| IBIS file stm32u3b5_3c5_wlcsp99_smps.ibs
[IBIS ver] 4.2
[File name] stm32u3b5_3c5_wlcsp99_smps.ibs
[File Rev] 0.1
[Date] 09-03-2026
[Source] Data Created at STMicroelectronics
[Notes]  File originated from ELDO simulations.
[Disclaimer]  This information is for modeling purpose only and is
   not guaranted. The information is subject to change without
   notice.
[Copyright] Copyright 2026 STMicroelectronics Inc.
|   Component stm32u3b5_3c5_wlcsp99_smps
[Component] stm32u3b5_3c5_wlcsp99_smps
[Manufacturer] STMicroelectronics
[Package]
| variable   typ   min   max
R_pkg  0  NA  NA
L_pkg  0  NA  NA
C_pkg  0  NA  NA
[Pin]   signal_name   model_name
A1  VDD  power
A3  PC11  io8_ft_100m_hslv
A5  PG9  io8_ft_100m_hslv
A7  VDDIO2  power
A9  PE2  io8_ft_100m
A11  VDD  power
B2  VSS  gnd
B4  PD2  io8_ft_100m_hslv
B6  VSS  gnd
B8  PB8  io8_ft_100m_hslv
B10  VSS  gnd
C1  VDDUSB  power
C3  PC10  io8_ft_100m_hslv
C5  PG10  io8_ft_100m_hslv
C7  PB3  io8_ft_100m_hslv
C9  PE3  io8_ft_100m_hslv
C11  VBAT  power
D2  PA14  io8_ft_100m
D4  PC12  io8_ft_100m_hslv
D6  PG13  io8_ft_100m_hslv
D8  PB9  io8_ft_100m_hslv
D10  PE6  io8_ft_100m
E1  PA12  io8usb_ft_phy
E3  PA15  io8_ft_100m
E5  PG11  io8_ft_100m_hslv
E7  PB4  io8_ft_100m_hslv
E9  PC13  io8_ft_100m_v33
E11  PC14-OSC32_IN  io_ft_tamp
F2  PA13  io8_ft_100m
F4  PA8  io8_ft_100m_hslv
F6  PG14  io8_ft_100m_hslv
F8  PH3-BOOT0  io8_ft_100m_hslv
F10  PE5  io8_ft_100m
G1  PA11  io8usb_ft_phy
G3  PA10  io8_ft_100m
G5  PG12  io8_ft_100m_hslv
G7  PB5  io8_ft_100m_hslv
G9  PE4  io8_ft_100m
G11  PC15-OSC32_OUT  io_ft_tamp
H2  PA9  io8_ft_100m
H4  PC9  io8_ft_100m_hslv
H6  PG15  io8_ft_100m_hslv
H8  PB7  io8_ft_100m_hslv
H10  NRST  ioreset_v33
J1  VDDIO2  power
J3  PC7  io8_ft_100m_hslv
J5  PC8  io8_ft_100m_hslv
J7  PB6  io8_ft_100m_hslv
J9  PC0  io8_ft_100m_hslv
J11  PH0-OSC_IN  io8_ft_100m
K2  VSS  gnd
K4  PG6  io8_ft_100m_hslv
K6  PC6  io8_ft_100m_hslv
K8  PC2  io8_ft_100m_hslv
K10  PC1  io8_ft_100m_hslv
L1  PG8  io8_ft_100m_hslv
L3  PG7  io8_ft_100m_hslv
L5  PG5  io8_ft_100m_hslv
L7  PA3  io8_ft_100m_hslv
L9  PC3  io8_ft_100m_hslv
L11  PH1-OSC_OUT  io8_ft_100m
M2  PG4  io8_ft_100m_hslv
M4  PG3  io8_ft_100m_hslv
M6  PE13  io8_ft_100m_hslv
M8  PA2  io8_ft_100m_hslv
M10  PA0  io8_ft_100m
N1  PG2  io8_ft_100m_hslv
N3  PB15  io8_ft_100m
N5  PB10  io8_ft_100m_hslv
N7  PA7  io8_ft_100m_hslv
N9  PA1  io8_ft_100m_hslv
N11  VREFP  nc
P2  PB13  io8_ft_100m_hslv
P4  PB14  io8_ft_100m_hslv
P6  PE12  io8_ft_100m_hslv
P8  PA6  io8_ft_100m_hslv
P10  VSSA_VREFM  nc
R1  PB12  io8_ft_100m_hslv
R3  VSSSMPS  nc
R5  PE15  io8_ft_100m_hslv
R7  PB2  io8_ft_100m_hslv
R9  PA5  io8_ft_100m
R11  VDDA  nc
T2  VSS  gnd
T4  PB11  io8_ft_100m_hslv
T6  PE11  io8_ft_100m_hslv
T8  PB1  io8_ft_100m_hslv
T10  PA4  io8_ft_100m_hslv
U1  VDD  power
U3  VDDSMPS  nc
U5  PE14  io8_ft_100m_hslv
U7  PE7  io8_ft_100m
U9  PB0  io8_ft_100m_hslv
U11  VDD  power
V2  VDD11  nc
V4  VLXSMPS  nc
V6  PE10  io8_ft_100m_hslv
V8  PE8  io8_ft_100m
V10  VSS  gnd
[Package Model]   42a-wlcsp-99-260114
[Pin Mapping]   pulldown_ref   pullup_ref   | Comment
A1  nc  vddio
A3  gndio  vddio
A5  gndio  vddio2
A7  nc  vddio2
A9  gndio  vddio
A11  nc  vddio
B2  gndio  nc
B4  gndio  vddio
B6  gndio  nc
B8  gndio  vddio
B10  gndio  nc
C1  nc  vddusb
C3  gndio  vddio
C5  gndio  vddio2
C7  gndio  vddio
C9  gndio  vddio
C11  nc  vsw
D2  gndio  vddio
D4  gndio  vddio
D6  gndio  vddio2
D8  gndio  vddio
D10  gndio  vddio
E1  gndio  vddusb  | Depending on IO usage
| E1  gndio  vddio  | Depending on IO usage
E3  gndio  vddio
E5  gndio  vddio2
E7  gndio  vddio
E9  gndio  vsw
E11  gndio  vsw
F2  gndio  vddio
F4  gndio  vddio
F6  gndio  vddio2
F8  gndio  vddio
F10  gndio  vddio
G1  gndio  vddusb  | Depending on IO usage
| G1  gndio  vddio  | Depending on IO usage
G3  gndio  vddio
G5  gndio  vddio2
G7  gndio  vddio
G9  gndio  vddio
G11  gndio  vsw
H2  gndio  vddio
H4  gndio  vddio
H6  gndio  vddio2
H8  gndio  vddio
H10  gndio  vddio
J1  nc  vddio2
J3  gndio  vddio
J5  gndio  vddio
J7  gndio  vddio
J9  gndio  vddio
J11  gndio  vddio
K2  gndio  nc
K4  gndio  vddio2
K6  gndio  vddio
K8  gndio  vddio
K10  gndio  vddio
L1  gndio  vddio2
L3  gndio  vddio2
L5  gndio  vddio2
L7  gndio  vddio
L9  gndio  vddio
L11  gndio  vddio
M2  gndio  vddio2
M4  gndio  vddio2
M6  gndio  vddio
M8  gndio  vddio
M10  gndio  vddio
N1  gndio  vddio2
N3  gndio  vddio
N5  gndio  vddio
N7  gndio  vddio
N9  gndio  vddio
N11  nc  nc
P2  gndio  vddio
P4  gndio  vddio
P6  gndio  vddio
P8  gndio  vddio
P10  nc  nc
R1  gndio  vddio
R3  nc  nc
R5  gndio  vddio
R7  gndio  vddio
R9  gndio  vddio
R11  nc  nc
T2  gndio  nc
T4  gndio  vddio
T6  gndio  vddio
T8  gndio  vddio
T10  gndio  vddio
U1  nc  vddio
U3  nc  nc
U5  gndio  vddio
U7  gndio  vddio
U9  gndio  vddio
U11  nc  vddio
V2  nc  nc
V4  nc  nc
V6  gndio  vddio
V8  gndio  vddio
V10  gndio  nc
|[Diff Pin]  inv_pin  vdiff  tdelay_typ  tdelay_min  tdelay_max
|E1  G1  NA  NA  NA  NA
[Model Selector] io8_ft_100m
io8_ft_100m_ls_1v2  "GPIO 100MHz - 5V tolerant - low speed - 1.2V range"
io8_ft_100m_ls_1v8  "GPIO 100MHz - 5V tolerant - low speed - 1.8V range"
io8_ft_100m_ls_3v3  "GPIO 100MHz - 5V tolerant - low speed - 3.3V range"
io8_ft_100m_ms_1v2  "GPIO 100MHz - 5V tolerant - med speed - 1.2V range"
io8_ft_100m_ms_1v8  "GPIO 100MHz - 5V tolerant - med speed - 1.8V range"
io8_ft_100m_ms_3v3  "GPIO 100MHz - 5V tolerant - med speed - 3.3V range"
io8_ft_100m_fs_1v2  "GPIO 100MHz - 5V tolerant - fast speed - 1.2V range"
io8_ft_100m_fs_1v8  "GPIO 100MHz - 5V tolerant - fast speed - 1.8V range"
io8_ft_100m_fs_3v3  "GPIO 100MHz - 5V tolerant - fast speed - 3.3V range"
io8_ft_100m_hs_1v2  "GPIO 100MHz - 5V tolerant - high speed - 1.2V range"
io8_ft_100m_hs_1v8  "GPIO 100MHz - 5V tolerant - high speed - 1.8V range"
io8_ft_100m_hs_3v3  "GPIO 100MHz - 5V tolerant - high speed - 3.3V range"
[Model Selector] io8_ft_100m_hslv
io8_ft_100m_ls_1v2  "GPIO 100MHz - 5V tolerant - low speed - 1.2V range"
io8_ft_100m_ls_1v8  "GPIO 100MHz - 5V tolerant - low speed - 1.8V range"
io8_ft_100m_ls_3v3  "GPIO 100MHz - 5V tolerant - low speed - 3.3V range"
io8_ft_100m_ms_1v2  "GPIO 100MHz - 5V tolerant - med speed - 1.2V range"
io8_ft_100m_ms_1v8  "GPIO 100MHz - 5V tolerant - med speed - 1.8V range"
io8_ft_100m_ms_3v3  "GPIO 100MHz - 5V tolerant - med speed - 3.3V range"
io8_ft_100m_fs_1v2  "GPIO 100MHz - 5V tolerant - fast speed - 1.2V range"
io8_ft_100m_fs_1v8  "GPIO 100MHz - 5V tolerant - fast speed - 1.8V range"
io8_ft_100m_fs_3v3  "GPIO 100MHz - 5V tolerant - fast speed - 3.3V range"
io8_ft_100m_hs_1v2  "GPIO 100MHz - 5V tolerant - high speed - 1.2V range"
io8_ft_100m_hs_1v8  "GPIO 100MHz - 5V tolerant - high speed - 1.8V range"
io8_ft_100m_hs_3v3  "GPIO 100MHz - 5V tolerant - high speed - 3.3V range"
io8_ft_100m_hslv_ls_1v2  "GPIO 100MHz low voltage optimization - 5V tolerant - low speed - 1.2V range"
io8_ft_100m_hslv_ls_1v8  "GPIO 100MHz low voltage optimization - 5V tolerant - low speed - 1.8V range"
io8_ft_100m_hslv_ls_2v5  "GPIO 100MHz low voltage optimization - 5V tolerant - low speed - 3.3V range"
io8_ft_100m_hslv_ms_1v2  "GPIO 100MHz low voltage optimization - 5V tolerant - med speed - 1.2V range"
io8_ft_100m_hslv_ms_1v8  "GPIO 100MHz low voltage optimization - 5V tolerant - med speed - 1.8V range"
io8_ft_100m_hslv_ms_2v5  "GPIO 100MHz low voltage optimization - 5V tolerant - med speed - 3.3V range"
io8_ft_100m_hslv_fs_1v2  "GPIO 100MHz low voltage optimization - 5V tolerant - fast speed - 1.2V range"
io8_ft_100m_hslv_fs_1v8  "GPIO 100MHz low voltage optimization - 5V tolerant - fast speed - 1.8V range"
io8_ft_100m_hslv_fs_2v5  "GPIO 100MHz low voltage optimization - 5V tolerant - fast speed - 3.3V range"
io8_ft_100m_hslv_hs_1v2  "GPIO 100MHz low voltage optimization - 5V tolerant - high speed - 1.2V range"
io8_ft_100m_hslv_hs_1v8  "GPIO 100MHz low voltage optimization - 5V tolerant - high speed - 1.8V range"
io8_ft_100m_hslv_hs_2v5  "GPIO 100MHz low voltage optimization - 5V tolerant - high speed - 3.3V range"
[Model Selector] io8_ft_100m_v33
io8_ft_100m_v33_ls_1v2  "GPIO_V33 100MHz - 5V tolerant - low speed - 1.2V range"
io8_ft_100m_v33_ls_1v8  "GPIO_V33 100MHz - 5V tolerant - low speed - 1.8V range"
io8_ft_100m_v33_ls_3v3  "GPIO_V33 100MHz - 5V tolerant - low speed - 3.3V range"
io8_ft_100m_v33_ms_1v2  "GPIO_V33 100MHz - 5V tolerant - med speed - 1.2V range"
io8_ft_100m_v33_ms_1v8  "GPIO_V33 100MHz - 5V tolerant - med speed - 1.8V range"
io8_ft_100m_v33_ms_3v3  "GPIO_V33 100MHz - 5V tolerant - med speed - 3.3V range"
io8_ft_100m_v33_fs_1v2  "GPIO_V33 100MHz - 5V tolerant - fast speed - 1.2V range"
io8_ft_100m_v33_fs_1v8  "GPIO_V33 100MHz - 5V tolerant - fast speed - 1.8V range"
io8_ft_100m_v33_fs_3v3  "GPIO_V33 100MHz - 5V tolerant - fast speed - 3.3V range"
io8_ft_100m_v33_hs_1v2  "GPIO_V33 100MHz - 5V tolerant - high speed - 1.2V range"
io8_ft_100m_v33_hs_1v8  "GPIO_V33 100MHz - 5V tolerant - high speed - 1.8V range"
io8_ft_100m_v33_hs_3v3  "GPIO_V33 100MHz - 5V tolerant - high speed - 3.3V range"
[Model Selector] io8usb_ft_phy
io8_ft_100m_ls_1v2  "GPIO 100MHz - 5V tolerant - low speed - 1.2V range"
io8_ft_100m_ls_1v8  "GPIO 100MHz - 5V tolerant - low speed - 1.8V range"
io8_ft_100m_ls_3v3  "GPIO 100MHz - 5V tolerant - low speed - 3.3V range"
io8_ft_100m_ms_1v2  "GPIO 100MHz - 5V tolerant - med speed - 1.2V range"
io8_ft_100m_ms_1v8  "GPIO 100MHz - 5V tolerant - med speed - 1.8V range"
io8_ft_100m_ms_3v3  "GPIO 100MHz - 5V tolerant - med speed - 3.3V range"
io8_ft_100m_fs_1v2  "GPIO 100MHz - 5V tolerant - fast speed - 1.2V range"
io8_ft_100m_fs_1v8  "GPIO 100MHz - 5V tolerant - fast speed - 1.8V range"
io8_ft_100m_fs_3v3  "GPIO 100MHz - 5V tolerant - fast speed - 3.3V range"
io8_ft_100m_hs_1v2  "GPIO 100MHz - 5V tolerant - high speed - 1.2V range"
io8_ft_100m_hs_1v8  "GPIO 100MHz - 5V tolerant - high speed - 1.8V range"
io8_ft_100m_hs_3v3  "GPIO 100MHz - 5V tolerant - high speed - 3.3V range"
io8usb_ft_phy_hs_3v3   "USB full speed"
io8usb_ft_phy_ls_3v3   "USB low speed"
[Model Selector] io_ft_tamp
io_ft_tamp_ls_1v2 "io8_ft tamp low speed @ 1.2V"
io_ft_tamp_ls_1v8 "io8_ft tamp low speed @ 1.8V"
io_ft_tamp_ls_3v3 "io8_ft tamp low speed @ 3.3V"
io_ft_tamp_ms_1v2 "io8_ft tamp med speed @ 1.2V"
io_ft_tamp_ms_1v8 "io8_ft tamp med speed @ 1.8V"
io_ft_tamp_ms_3v3 "io8_ft tamp med speed @ 3.3V"
io_ft_tamp_fs_1v2 "io8_ft tamp fast speed @ 1.2V"
io_ft_tamp_fs_1v8 "io8_ft tamp fast speed @ 1.8V"
io_ft_tamp_fs_3v3 "io8_ft tamp fast speed @ 3.3V"
io_ft_tamp_hs_1v2 "io8_ft tamp high speed @ 1.2V"
io_ft_tamp_hs_1v8 "io8_ft tamp high speed @ 1.8V"
io_ft_tamp_hs_3v3 "io8_ft tamp high speed @ 3.3V"
[Model Selector] ioreset_v33
ioreset_v33_1v2 "Reset PAD. 5V tolerant. 1.2V range"
ioreset_v33_1v8 "Reset PAD. 5V tolerant. 1.8V range"
ioreset_v33_3v3 "Reset PAD. 5V tolerant. 3.3V range"
[Define Package Model]  42a-wlcsp-99-260114
[Manufacturer]  Unknown
[OEM]  Unknown
[Description]  None
[Number Of Pins]  91
[Pin Numbers]
| Pin Num   Terminal Name
H10 | NRST
M10 | PA0
N9 | PA1
M8 | PA2
L7 | PA3
T10 | PA4
R9 | PA5
P8 | PA6
N7 | PA7
F4 | PA8
H2 | PA9
G3 | PA10
G1 | PA11
E1 | PA12
F2 | PA13
D2 | PA14
E3 | PA15
U9 | PB0
T8 | PB1
R7 | PB2
C7 | PB3
E7 | PB4
G7 | PB5
J7 | PB6
H8 | PB7
B8 | PB8
D8 | PB9
N5 | PB10
T4 | PB11
R1 | PB12
P2 | PB13
P4 | PB14
N3 | PB15
J9 | PC0
K10 | PC1
K8 | PC2
L9 | PC3
K6 | PC6
J3 | PC7
J5 | PC8
H4 | PC9
C3 | PC10
A3 | PC11
D4 | PC12
E9 | PC13
E11 | PC14-OSC32_IN
G11 | PC15-OSC32_OUT
B4 | PD2
A9 | PE2
C9 | PE3
G9 | PE4
F10 | PE5
D10 | PE6
U7 | PE7
V8 | PE8
V6 | PE10
T6 | PE11
P6 | PE12
M6 | PE13
U5 | PE14
R5 | PE15
N1 | PG2
M4 | PG3
M2 | PG4
L5 | PG5
K4 | PG6
L3 | PG7
L1 | PG8
A5 | PG9
C5 | PG10
E5 | PG11
G5 | PG12
D6 | PG13
F6 | PG14
H6 | PG15
J11 | PH0-OSC_IN
L11 | PH1-OSC_OUT
F8 | PH3-BOOT0
V2 | VDD11
C11 | VBAT
A1 | VDD
R11 | VDDA
J1 | VDDIO2
A7 | VDDIO2
U3 | VDDSMPS
C1 | VDDUSB
V4 | VLXSMPS
N11 | VREFP
B2 | VSS
P10 | VSSA_VREFM
R3 | VSSSMPS
|[Merged Pins]  A1
|A11  |  VDD
|U1  |  VDD
|U11  |  VDD
|[Merged Pins]  B2
|B6  |  VSS
|B10  |  VSS
|K2  |  VSS
|T2  |  VSS
|V10  |  VSS
[Model Data]
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[End Model Data]
[End Package Model]
|End [Component]
| Models and submodels in the file (53): io8_ft_100m_fs_1v2 (I/O), io8_ft_100m_fs_1v8 (I/O), io8_ft_100m_fs_3v3 (I/O), io8_ft_100m_hs_1v2 (I/O), io8_ft_100m_hs_1v8 (I/O), io8_ft_100m_hs_3v3 (I/O), io8_ft_100m_hslv_fs_1v2 (I/O), io8_ft_100m_hslv_fs_1v8 (I/O), io8_ft_100m_hslv_fs_2v5 (I/O), io8_ft_100m_hslv_hs_1v2 (I/O), io8_ft_100m_hslv_hs_1v8 (I/O), io8_ft_100m_hslv_hs_2v5 (I/O), io8_ft_100m_hslv_ls_1v2 (I/O), io8_ft_100m_hslv_ls_1v8 (I/O), io8_ft_100m_hslv_ls_2v5 (I/O), io8_ft_100m_hslv_ms_1v2 (I/O), io8_ft_100m_hslv_ms_1v8 (I/O), io8_ft_100m_hslv_ms_2v5 (I/O), io8_ft_100m_ls_1v2 (I/O), io8_ft_100m_ls_1v8 (I/O), io8_ft_100m_ls_3v3 (I/O), io8_ft_100m_ms_1v2 (I/O), io8_ft_100m_ms_1v8 (I/O), io8_ft_100m_ms_3v3 (I/O), io8_ft_100m_v33_fs_1v2 (I/O), io8_ft_100m_v33_fs_1v8 (I/O), io8_ft_100m_v33_fs_3v3 (I/O), io8_ft_100m_v33_hs_1v2 (I/O), io8_ft_100m_v33_hs_1v8 (I/O), io8_ft_100m_v33_hs_3v3 (I/O), io8_ft_100m_v33_ls_1v2 (I/O), io8_ft_100m_v33_ls_1v8 (I/O), io8_ft_100m_v33_ls_3v3 (I/O), io8_ft_100m_v33_ms_1v2 (I/O), io8_ft_100m_v33_ms_1v8 (I/O), io8_ft_100m_v33_ms_3v3 (I/O), io8usb_ft_phy_hs_3v3 (I/O), io8usb_ft_phy_ls_3v3 (I/O), io_ft_tamp_fs_1v2 (I/O), io_ft_tamp_fs_1v8 (I/O), io_ft_tamp_fs_3v3 (I/O), io_ft_tamp_hs_1v2 (I/O), io_ft_tamp_hs_1v8 (I/O), io_ft_tamp_hs_3v3 (I/O), io_ft_tamp_ls_1v2 (I/O), io_ft_tamp_ls_1v8 (I/O), io_ft_tamp_ls_3v3 (I/O), io_ft_tamp_ms_1v2 (I/O), io_ft_tamp_ms_1v8 (I/O), io_ft_tamp_ms_3v3 (I/O), ioreset_v33_1v2 (I/O_open_drain), ioreset_v33_1v8 (I/O_open_drain), ioreset_v33_3v3 (I/O_open_drain)
